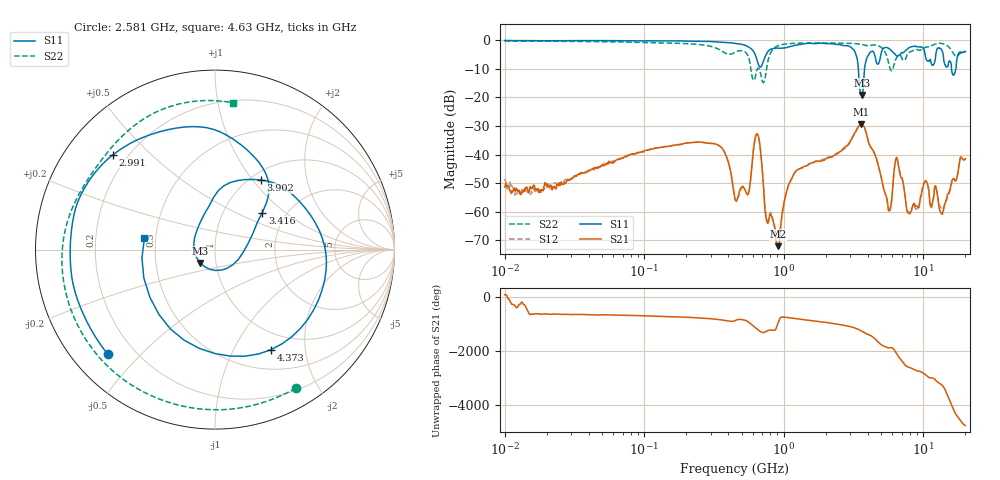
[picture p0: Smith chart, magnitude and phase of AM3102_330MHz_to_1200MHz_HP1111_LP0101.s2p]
! Date/Time: Tue, Sep 11, 2018 5:24 PM
! Network Analyzer: Agilent Technologies E8362B Rev: A.07.50.63
! Sweep from 0.010 to 20.000 GHz, 1601 Points, Sweep Type: LOG
! Power Supply: 4.949 V, 0.001 A
# Hz S DB R 50
!freq MagS11 AngS11 MagS21 AngS21 MagS12 AngS12 MagS22 AngS22
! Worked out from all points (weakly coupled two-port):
!   1601 points, 10 MHz to 20 GHz, reference 50 ohm
!   highest |S21| = -29.41 dB at 3.565 GHz (marker M1); lowest = -72.1 dB at 907.7 MHz (marker M2)
!   lowest |S11| = -19.1 dB at 3.617 GHz (marker M3), VSWR 1.25, Z = 41.9 - j6.28 ohm
!   |S11| at or under -10 dB: 3.421 GHz to 3.787 GHz (365.6 MHz wide, 10.1 % of centre); 15.91 GHz to 17.11 GHz (1.2 GHz wide, 7.27 % of centre)
!   |S22| runs from -14.8 to -0.2 dB; largest |S21 - S12| = 0.0065
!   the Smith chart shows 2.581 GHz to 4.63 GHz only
!   S11 on the Smith chart (normalised r, x): 2.581 GHz: 0.11, -0.40; 2.991 GHz: 0.15, +0.39; 3.416 GHz: 1.52, +0.70; 3.902 GHz: 1.11, +1.10; 4.373 GHz: 0.75, -1.42; 4.63 GHz: 0.43, +0.07
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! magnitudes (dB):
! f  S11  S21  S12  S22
! 10 MHz  0.0  -51.4  -48.6  -0.2
! 35.55 MHz  -0.1  -46.5  -46.6  -0.4
! 126.4 MHz  -0.2  -37.7  -37.6  -0.8
! 341.1 MHz  -0.6  -36.8  -36.7  -3.1
! 447.2 MHz  -1.0  -55.5  -55.5  -4.2
! 647.8 MHz  -7.4  -32.9  -32.9  -9.9
! 750.6 MHz  -4.8  -62.9  -62.1  -10.3
! 907.7 MHz  -2.7  -72.1  -69.4  -1.9
! 1.59 GHz  -1.1  -42.9  -42.9  -0.9
! 2.581 GHz  -1.6  -38.8  -38.8  -1.0
! 2.991 GHz  -2.2  -35.4  -35.3  -1.0
! 3.416 GHz  -9.5  -30.2  -30.5  -1.2
! 3.565 GHz  -18.7  -29.4  -29.4  -1.3
! 3.617 GHz  -19.1  -29.5  -29.3  -1.4
! 3.902 GHz  -6.7  -32.6  -32.6  -1.8
! 4.373 GHz  -3.9  -38.7  -38.6  -1.6
! 4.63 GHz  -8.0  -41.7  -41.8  -1.7
! 5.652 GHz  -2.8  -59.6  -60.0  -8.2
! 6.426 GHz  -5.4  -41.0  -41.4  -6.1
! 7.845 GHz  -2.7  -60.5  -60.0  -4.3
! 13.48 GHz  -3.3  -60.6  -59.0  -1.1
! 20 GHz  -4.0  -41.5  -42.0  -3.8
